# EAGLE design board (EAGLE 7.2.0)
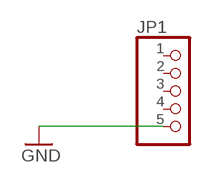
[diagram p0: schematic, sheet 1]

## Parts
JP1  PINHD-1X5_2.54  [1X05]

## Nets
GND: JP1.5
Unconnected: JP1.1 JP1.2 JP1.3 JP1.4

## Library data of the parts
JP1 = pinhead:PINHD-1X5: PIN HEADER

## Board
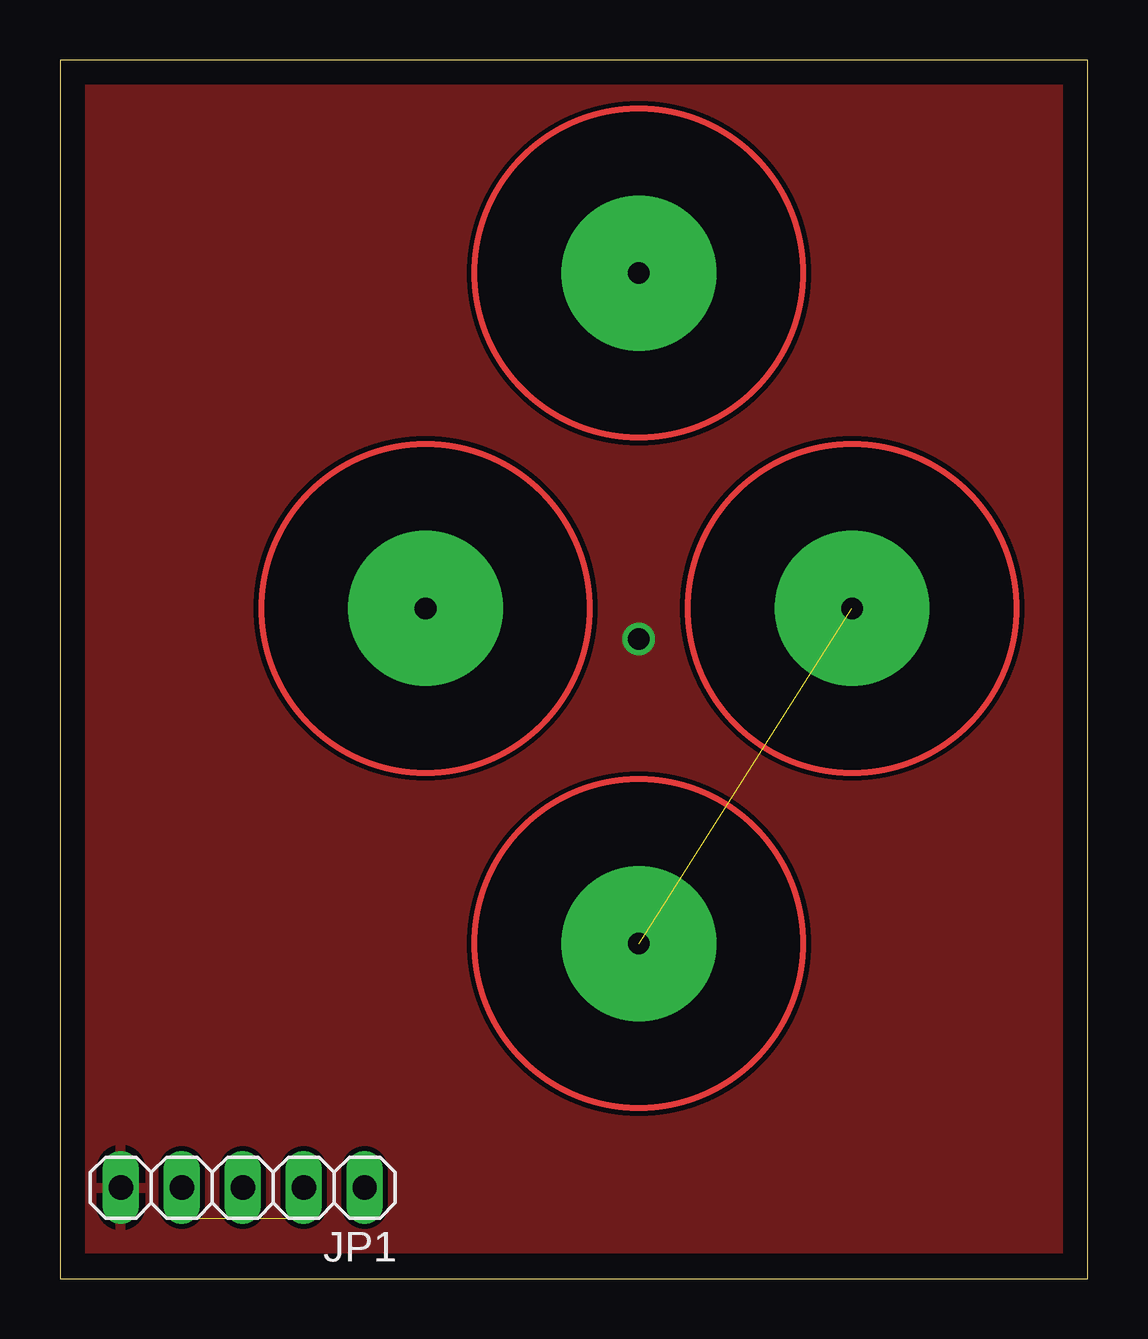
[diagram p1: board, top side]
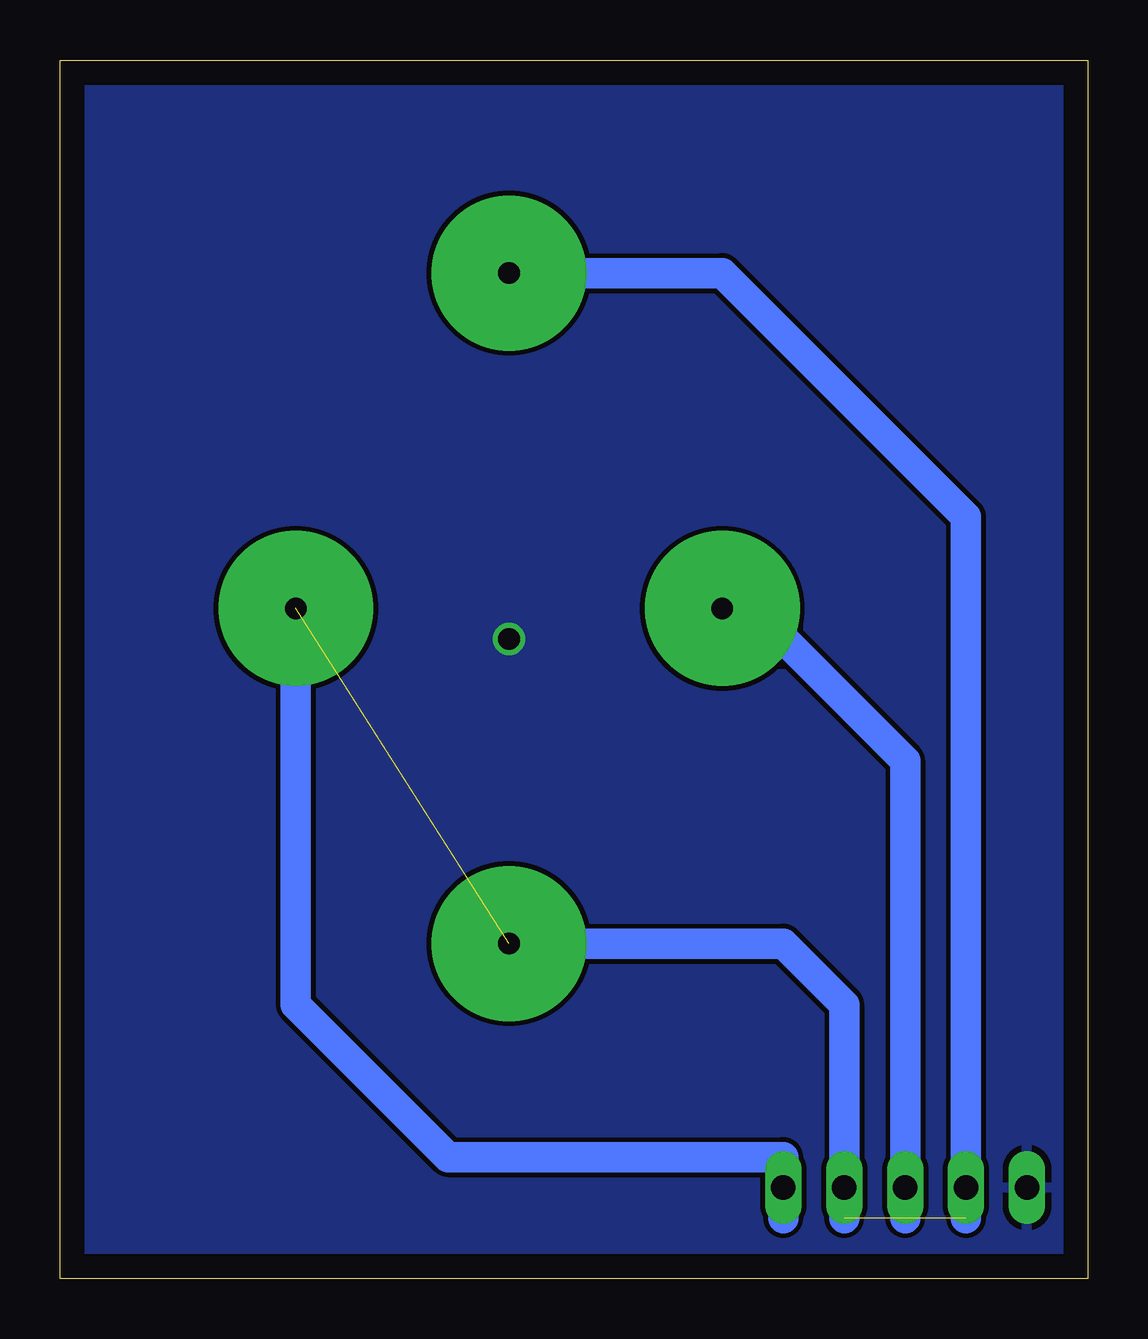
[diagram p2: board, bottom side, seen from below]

Size 42.85 x 50.79 mm. Coordinates in mm from the lower left corner, seen from the top.
Outline: 0,0 42.85,0 42.85,50.79 0,50.79 0,0
Copper layers (1*16): Top 0.035mm / dielectric 1.5mm / Bottom 0.035mm
Design rules "default": minimum track width 10mil, minimum drill 24mil, track to track 8mil, track to pad 8mil, pad to pad 8mil, via to via 8mil, smd to smd 8mil, copper to edge 40mil, drill to drill 8mil, minimum pad ring 10mil, minimum via ring 8mil, stop-mask expansion 4mil, vias tented up to drill 0mil, thermal gap 10mil

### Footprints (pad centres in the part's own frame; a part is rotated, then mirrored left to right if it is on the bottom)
1X05 = drill 1.016 long: 1 -5.08,0; 2 -2.54,0; 3 0,0; 4 2.54,0; 5 5.08,0

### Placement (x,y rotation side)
JP1  7.62,3.81 180 top

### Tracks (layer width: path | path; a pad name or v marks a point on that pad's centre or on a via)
GND  (via drill 0.9 pad 1.27)
  other vias: 24.13,26.67
  pour Top: 0,1.27 64.77,1.27 64.77,58.42 0,58.42
  pour Bottom: 0,1.27 0,59.69 1.27,60.96 66.04,60.96 66.04,0 1.27,0
N$1
  Bottom 1.27: 33.02,27.94 33.02,11.43 26.67,5.08 12.7,5.08 12.7,2.54
N$4  (via drill 0.9 pad 6.45)  (3 unrouted)
  Bottom 1.27: v15.24,27.94 13.97,27.94 7.62,21.59 7.62,2.54 | v24.13,41.91 15.24,41.91 5.08,31.75 5.08,2.54 | v24.13,13.97 12.7,13.97 10.16,11.43 10.16,2.54
  other vias: 33.02,27.94
(copper drawn outside any net)
  shapes: Top circle x4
